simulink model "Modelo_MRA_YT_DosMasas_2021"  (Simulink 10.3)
settings: Solver=VariableStepAuto  StartTime=0.0  StopTime=30  RelTol=1e-3
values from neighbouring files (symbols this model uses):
  b1 = 2    [Modelo_MRA_2DOF.m]
  b2 = 1.5    [Modelo_MRA_2DOF.m]
  k1 = 50    [Modelo_MRA_2DOF.m]
  k2 = 30    [Modelo_MRA_2DOF.m]
  m1 = 10    [Modelo_MRA_2DOF.m]
  m2 = 5    [Modelo_MRA_2DOF.m]

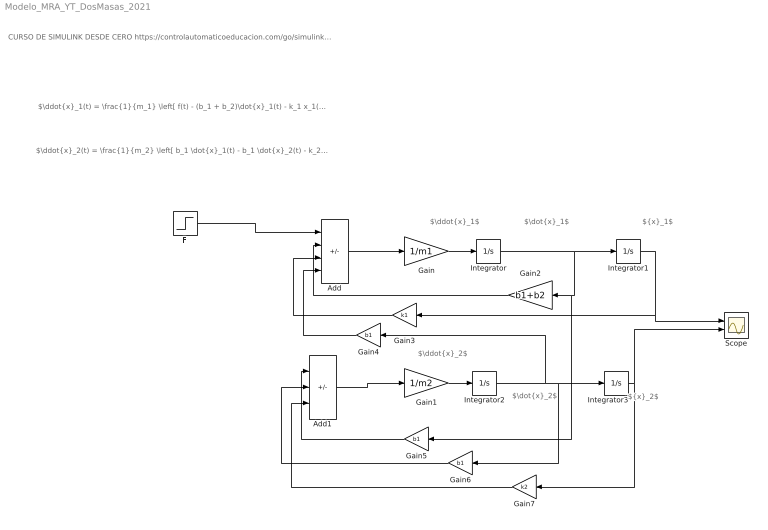
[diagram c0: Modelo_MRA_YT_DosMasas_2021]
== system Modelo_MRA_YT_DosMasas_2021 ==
  note: $\ddot{x}_1$
  note: $\ddot{x}_1(t) = \frac{1}{m_1} \left[ f(t) - (b_1 + b_2)\dot{x}_1(t) - k_1 x_1(t) + b_1 \dot{x}_2(t) \right]$
  note: CURSO DE SIMULINK DESDE CERO https://controlautomaticoeducacion.com/go/simulink-cupon/
  note: $\ddot{x}_2(t) = \frac{1}{m_2} \left[ b_1 \dot{x}_1(t) - b_1 \dot{x}_2(t) - k_2 x_2(t) \right]$
  note: $\ddot{x}_2$
  note: $\dot{x}_1$
  note: ${x}_1$
  note: $\dot{x}_2$
  note: ${x}_2$
  Add : Sum  Inputs=+--+
  Add1 : Sum  Inputs=+--
  F : Step  Time=0  SampleTime=0
  Gain : Gain  Gain=1/m1
  Gain1 : Gain  Gain=1/m2
  Gain2 : Gain  Gain=b1+b2
  Gain3 : Gain  Gain=k1
  Gain4 : Gain  Gain=b1
  Gain5 : Gain  Gain=b1
  Gain6 : Gain  Gain=b1
  Gain7 : Gain  Gain=k2
  Integrator{,1..3} (4 alike) : Integrator
  Scope : Scope  NumInputPorts=2
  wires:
  Integrator/1 -> Gain5/1, Gain2/1, Integrator1/1
  Integrator2/1 -> Gain4/1, Gain6/1, Integrator3/1
  Gain/1 -> Integrator/1
  Gain1/1 -> Integrator2/1
  Add/1 -> Gain/1
  F/1 -> Add/1
  Gain2/1 -> Add/2
  Integrator1/1 -> Scope/1, Gain3/1
  Gain3/1 -> Add/3
  Gain4/1 -> Add/4
  Gain5/1 -> Add1/1
  Gain6/1 -> Add1/2
  Integrator3/1 -> Gain7/1, Scope/2
  Gain7/1 -> Add1/3
  Add1/1 -> Gain1/1
